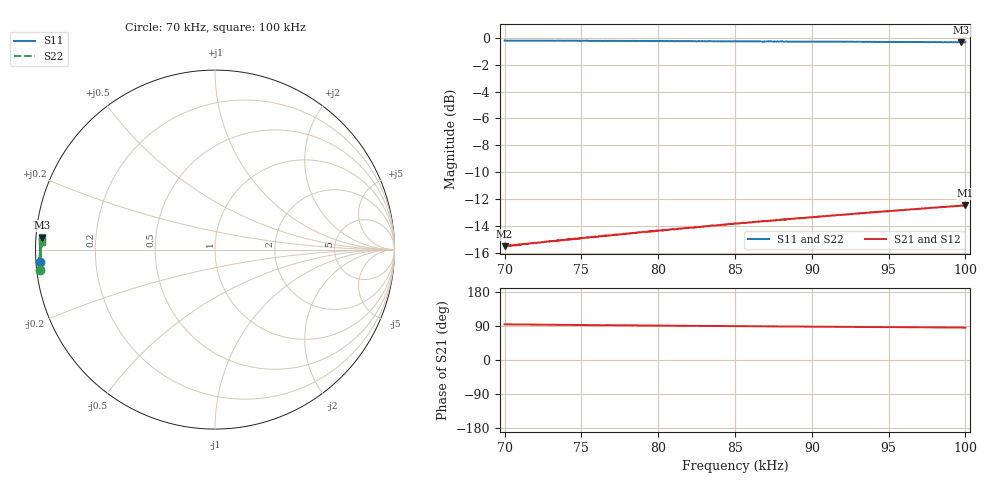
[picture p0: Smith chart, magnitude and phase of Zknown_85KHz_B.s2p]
!Keysight Technologies N9928A: A.12.01
!Date: Monday, January 30, 2023
!Model: N9928A
!Serial: MY58311550
!Caliblation kit: 85033D 3.5mm Calibration Kit
!DUT Connector Gender Port1: male
!DUT Connector Gender Port2: female
!S2P File: Measurements:S11,S21,S12,S22:
# Hz S DB R 50
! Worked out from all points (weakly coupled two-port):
!   1001 points, 70 kHz to 100 kHz, reference 50 ohm
!   highest |S21| = -12.48 dB at 99.97 kHz (marker M1); lowest = -15.5 dB at 70 kHz (marker M2)
!   lowest |S11| = -0.3 dB at 99.73 kHz (marker M3), VSWR 54.03, Z = 0.926 + j1.74 ohm
!   |S11| at or under -10 dB: nowhere
!   |S22| runs from -0.3 to -0.2 dB; largest |S21 - S12| = 0.0022
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70000  -0.18 -175.8  -15.53 94.1  -15.56 94.0  -0.19 -173.4
70270  -0.19 -175.9  -15.50 93.9  -15.47 93.8  -0.18 -173.5
70840  -0.19 -176.1  -15.42 93.8  -15.46 93.6  -0.19 -173.8
71170  -0.19 -176.3  -15.35 93.6  -15.37 93.6  -0.19 -173.9
71380  -0.20 -176.3  -15.36 93.8  -15.40 93.3  -0.18 -174.0
72130  -0.20 -176.5  -15.27 93.5  -15.29 93.5  -0.18 -174.2
72460  -0.19 -176.7  -15.22 93.4  -15.25 93.2  -0.19 -174.4
73330  -0.21 -176.9  -15.12 92.9  -15.14 92.8  -0.18 -174.6
75010  -0.20 -177.4  -14.93 92.3  -14.96 92.3  -0.21 -175.2
77680  -0.22 -178.3  -14.64 91.4  -14.63 91.6  -0.21 -176.1
80020  -0.22 -179.0  -14.37 90.7  -14.40 90.8  -0.21 -176.9
81280  -0.23 -179.3  -14.23 90.6  -14.25 90.6  -0.22 -177.3
81820  -0.23 -179.5  -14.18 90.2  -14.20 90.3  -0.22 -177.5
85000  -0.24 179.7  -13.83 89.4  -13.88 89.5  -0.23 -178.4
88300  -0.26 178.8  -13.55 88.4  -13.54 88.6  -0.26 -179.3
88840  -0.26 178.6  -13.48 88.4  -13.50 88.4  -0.26 -179.5
89230  -0.26 178.6  -13.42 88.4  -13.46 88.3  -0.26 -179.6
90010  -0.27 178.4  -13.38 88.1  -13.38 88.1  -0.26 -179.8
95020  -0.29 177.1  -12.92 86.8  -12.92 86.8  -0.28 178.8
99730  -0.32 176.0  -12.50 85.6  -12.54 85.7  -0.31 177.7
99970  -0.31 176.0  -12.48 85.5  -12.48 85.6  -0.32 177.6
100000  -0.31 176.0  -12.48 85.5  -12.50 85.6  -0.31 177.6
